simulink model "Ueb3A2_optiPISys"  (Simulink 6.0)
settings: Solver=ode45  StartTime=0.0  StopTime=10.0  RelTol=1e-3
libraries: cstblocks x2

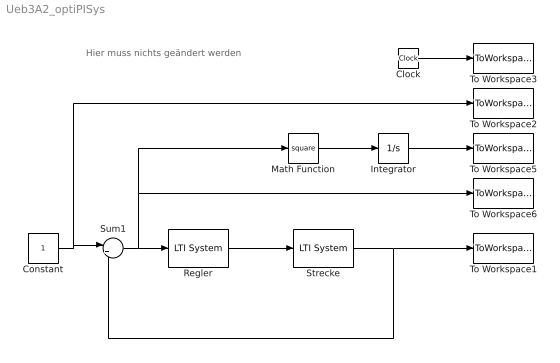
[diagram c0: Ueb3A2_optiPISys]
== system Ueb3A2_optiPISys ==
  note: Hier muss nichts geändert werden
  Clock : Clock
  Constant : Constant  Value=1  SampleTime=inf
  Integrator : Integrator  ExternalReset=none  InitialConditionSource=internal  InitialCondition=0  LimitOutput=off  UpperSaturationLimit=inf  LowerSaturationLimit=-inf  ShowSaturationPort=off  ShowStatePort=off  AbsoluteTolerance=auto
  Math Function : Math  Operator=square  OutputSignalType=auto  SampleTime=-1
  Regler : cstblocks/LTI System  sys=C  IC=[]
  Strecke : cstblocks/LTI System  sys=P  IC=[]
  Sum1 : Sum  Inputs=|+-  SaturateOnIntegerOverflow=on  SampleTime=-1
  To Workspace1 : ToWorkspace  VariableName=y  SampleTime=0.05  SaveFormat=Array
  To Workspace2 : ToWorkspace  VariableName=r  SampleTime=0.05  SaveFormat=Array
  To Workspace3 : ToWorkspace  VariableName=t  SampleTime=0.05  SaveFormat=Array
  To Workspace5 : ToWorkspace  VariableName=Je2  SampleTime=0.05  SaveFormat=Array
  To Workspace6 : ToWorkspace  VariableName=e  SampleTime=0.05  SaveFormat=Array
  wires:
  Strecke/1 -> To Workspace1/1, Sum1/2
  Constant/1 -> Sum1/1, To Workspace2/1
  Sum1/1 -> Regler/1, Math Function/1, To Workspace6/1
  Regler/1 -> Strecke/1
  Clock/1 -> To Workspace3/1
  Math Function/1 -> Integrator/1
  Integrator/1 -> To Workspace5/1
